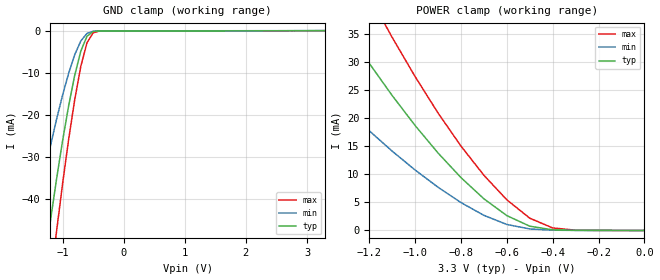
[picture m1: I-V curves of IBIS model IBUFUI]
| IBIS file ibufui.ibs created by s2ibis2 version 1.1
| North Carolina State University Electronics Research Laboratory  1995
[IBIS ver]   2.1
[File name]   ibufui.ibs
[File Rev]   1.0
[Date]   Thursday, March 30, 2000
[Source]   From silicon level SPICE at TOSHIBA.
[Notes]   This model does not include the values of Package Model
[Disclaimer]   None.
[Copyright]   Copyright(C) TOSHIBA Corp. 1996-2000. All Rights Reserved
|   Component TC260C
[Component]   TC260C
[Manufacturer]   TOSHIBA
[Package]
| variable   typ   min   max
R_pkg   1.0000f   NA   NA
L_pkg   1.0000fH   NA   NA
C_pkg   1.0000fF   NA   NA
[Pin]  signal_name   model_name   R_pin   L_pin   C_pin
A   A   IBUFUI
VDDS   VDDS   POWER
VSS   VSS   GND
| Models and submodels in the file (1): IBUFUI (Input)
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|   Model IBUFUI
[Model]   IBUFUI
Model_type   Input
Polarity   Non-Inverting
Vinl =   0.6600V
Vinh =   2.6400V
C_comp   4.3000pF   NA   NA
|Variable   typ   min   max
[Voltage range]  3.3   3.0   3.6
[Temperature Range]   25.0000   100.0000   0.000
[POWER Clamp Reference]   3.3000V   3.0000V   3.6000V
[GND Clamp Reference]   0.000V   0.000V   0.000V
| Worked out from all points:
|   GND clamp passes 1 mA (typ) near -0.57 V on its own axis
|   POWER clamp passes 1 mA (typ) near -0.51 V on its own axis
[GND_clamp]
| voltage   I(typ)   I(min)   I(max)
-3.3V     -292.9mA   -217.9mA   -337.6mA
-1.5V     -78.02mA   -49.1mA    -99.03mA
-1.3V     -55.93mA   -34.39mA   -72.82mA
-1.2V     -45.48mA   -27.6mA    -60.2mA
-1.1V     -35.57mA   -21.25mA   -48.06mA
-900mV    -17.92mA   -10.17mA   -25.93mA
-800mV    -10.62mA   -5.728mA   -16.42mA
-700mV    -4.847mA   -2.443mA   -8.473mA
-600mV    -1.357mA   -679.2uA   -2.912mA
-500mV    -225.1uA   -138.4uA   -522.2uA
-400mV    -68.02uA   -43.8uA    -112uA
3.3V      153.9pA    14.42uA    -16.89uA
[POWER_clamp]
| voltage   I(typ)   I(min)   I(max)
-3.3V     189.3mA    136.1mA    229.5mA
-1.7V     62.67mA    39.14mA    83.1mA
-1.6V     55.64mA    34.47mA    74.42mA
-1.3V     35.82mA    21.61mA    49.54mA
-1.2V     29.75mA    17.75mA    41.78mA
-1.1V     24.02mA    14.12mA    34.37mA
-900mV    13.79mA    7.692mA    20.91mA
-800mV    9.41mA     4.966mA    15.02mA
-600mV    2.644mA    1.069mA    5.459mA
-500mV    763.5uA    269.3uA    2.188mA
-400mV    115.4uA    51.5uA     450.7uA
0V        153.9pA    711.8pA    166.4pA
